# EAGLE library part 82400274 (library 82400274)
TVS Diode Array WE-TVS 4-Ch+VDD 5V SC70 Wurth Elektronik 82400274, Quad Uni-Directional TVS Diode Array, 6-Pin SC-70 Source: Datasheet
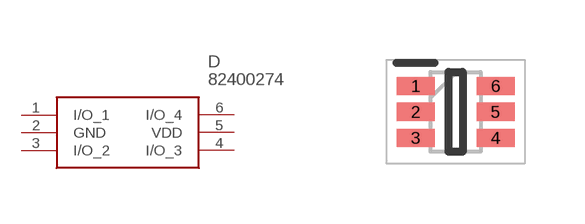
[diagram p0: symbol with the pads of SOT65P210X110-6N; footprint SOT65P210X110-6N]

Designator prefix D

## 82400274 (Description: TVS Diode Array WE-TVS 4-Ch+VDD 5V SC70 Wurth Elektronik 82400274, Quad Uni-Directional TVS Diode Array, 6-Pin SC-70; Height: 1.1mm; Manufacturer_Name: Wurth Elektronik; Manufacturer_Part_Number: 82400274; Mouser_Part_Number: 710-82400274; Mouser_Price-Stock: https://www.mouser.co.uk/ProductDetail/Wurth-Elektronik/82400274?qs=2kOmHSv6VfQD871MY%252BLLLQ%3D%3D)  [SOT65P210X110-6N]
1  I/O_1
2  GND
3  I/O_2
4  I/O_3
5  VDD
6  I/O_4

## Footprint SOT65P210X110-6N (pad centres in mm)
SC70-6L
smd 0.95 x 0.45: 1 -1,0.65; 2 -1,0; 3 -1,-0.65; 4 1,-0.65; 5 1,0; 6 1,0.65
